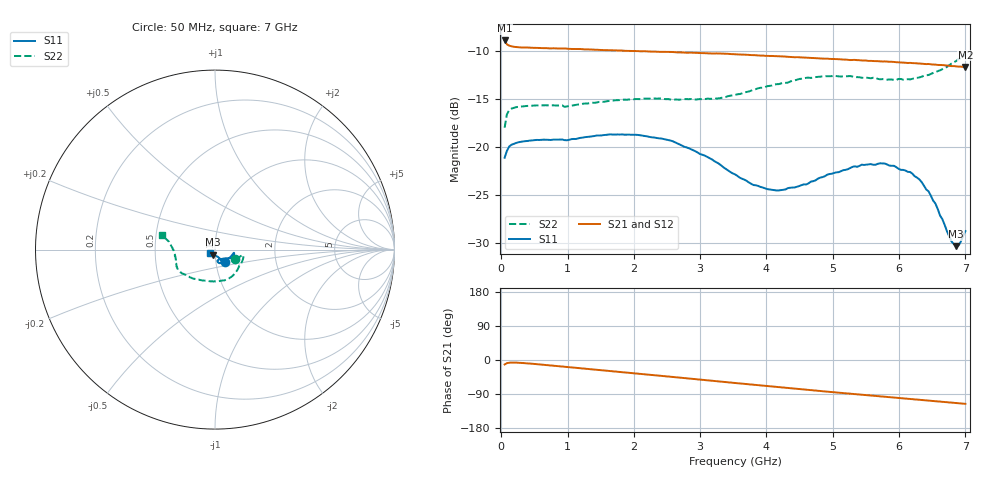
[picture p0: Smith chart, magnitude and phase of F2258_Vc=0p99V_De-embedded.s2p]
! Integrated Device Technology
! Corporate Headquarters
! 6024 Silver Creek Valley Road
! San Jose, CA 95138  USA
! Phone:  1-408-284-8200
! Toll Free:  1-800-223-1366
! Webpage:  http://www.idt.com/
! Timing and RF Division
! 515 Groton Road, Suite 102
! Westford, MA 01886-6024
! Device:  F2258
! Description: Voltage Variable RF Attenuator
! Frequency:  50.0 -  6000.00 MHz
! Package:  3x3 mm Thin QFN Plastic Package: 16 pin
! Ports:  2 RF, 2 DC
!  Pin  1  = NC
!  Pin  2  = NC
!  Pin  3  = RF2  = Port 2
!  Pin  4  = GND
!  Pin  5  = Vdd
!  Pin  6  = NC
!  Pin  7  = VCTRL
!  Pin  8  = NC
!  Pin  9  = GND
!  Pin 10  = RF1  = Port 1
!  Pin 11  = NC
!  Pin 12  = NC
!  Pin 13  = NC
!  Pin 14  = NC
!  Pin 15  = NC
!  Pin 16  = NC
! Vcntrl:  0.990 Volts
! Vdd:  +3.300 Volts
! Current:  1.155 mA
! Data:  The device was measured on a the F2258 evaluation board which has
!  individual transmission lines to the RF pins.  Data was collected
!  using a calibrated network analyzer.  The evaluation board was
!  de-embedded using a TRL calibration technique.
!  The reference plane is the edge of the package pin.
! Misc:  SN 10
!  Action Tracker AT0285
! Date Measured:  2014-12-10
! Date:  2016-01-13  MJV
! Note:
!  Integrated Device Technology supplies this data as a sample of measured
!  data at the package pin for this product.  Your particular data for this
!  product may vary.
!  Data was taken at 25 degrees C.
!  Integrated Device Technology reserves the right to change this data at anytime.
!Freq_(GHz)  S11M_(dB)  S11P_(deg)  S21M_(dB)  S21P_(deg)  S12M_(dB)  S12P_(deg)  S22M_(dB)  S22P_(deg)
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# GHz S dB R 50
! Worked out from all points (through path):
!   201 points, 50 MHz to 7 GHz, reference 50 ohm
!   highest |S21| = -8.88 dB at 50 MHz (marker M1); lowest = -11.6 dB at 7 GHz (marker M2)
!   group delay of S21, straight-line fit = 45.2 ps
!   lowest |S11| = -30.3 dB at 6.861 GHz (marker M3), VSWR 1.06, Z = 49 - j2.82 ohm
!   |S11| at or under -10 dB: start of sweep to end of sweep
!   |S22| runs from -18.0 to -10.3 dB; largest |S21 - S12| = 0.00099
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0.05  -21.12 -49.4  -8.88 -11.8  -8.86 -11.7  -17.99 -25.4
0.08475  -20.39 -24.8  -9.28 -8.4  -9.28 -8.4  -16.58 -13.9
0.1195  -19.94 -16.7  -9.42 -7.2  -9.43 -7.2  -16.15 -11.4
0.189  -19.66 -11.6  -9.54 -6.8  -9.53 -6.8  -15.91 -10.9
1.2315  -19.01 -19.5  -9.79 -22.4  -9.81 -22.4  -15.48 -41.3
1.82225  -18.68 -22.9  -9.93 -32.1  -9.94 -32.1  -15.06 -57.2
2.37825  -19.09 -25.0  -10.06 -41.3  -10.06 -41.3  -14.93 -72.5
2.58675  -19.39 -26.8  -10.08 -44.8  -10.09 -44.8  -15.08 -78.6
3.07325  -20.91 -32.2  -10.20 -53.0  -10.20 -53.0  -14.99 -96.3
3.525  -22.84 -43.4  -10.32 -60.7  -10.31 -60.7  -14.56 -114.5
3.803  -23.96 -55.0  -10.40 -65.4  -10.39 -65.4  -14.02 -125.1
4.1505  -24.53 -67.6  -10.52 -71.2  -10.53 -71.1  -13.44 -135.4
4.7065  -23.56 -77.7  -10.72 -80.2  -10.72 -80.2  -12.75 -148.0
5.43625  -21.84 -70.2  -10.96 -91.7  -10.96 -91.6  -12.77 -159.4
5.85325  -21.93 -62.6  -11.10 -98.2  -11.10 -98.2  -12.95 -167.9
6.166  -22.60 -59.9  -11.22 -103.1  -11.22 -103.1  -12.94 -175.2
6.33975  -23.65 -59.2  -11.30 -105.8  -11.30 -105.9  -12.66 179.9
6.54825  -25.90 -64.3  -11.40 -109.0  -11.39 -109.1  -12.18 174.7
6.7915  -29.86 -93.1  -11.55 -112.6  -11.54 -112.6  -11.28 168.7
6.861  -30.34 -108.6  -11.58 -113.7  -11.56 -113.7  -11.02 167.5
6.89575  -30.28 -118.9  -11.61 -114.2  -11.60 -114.2  -10.83 166.8
7  -28.77 -144.6  -11.64 -115.7  -11.64 -115.8  -10.34 164.8
